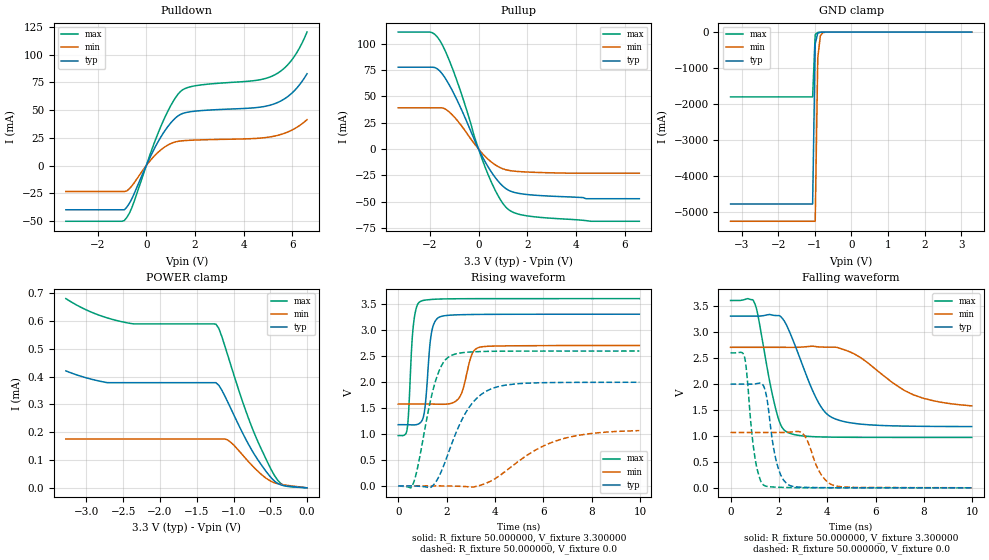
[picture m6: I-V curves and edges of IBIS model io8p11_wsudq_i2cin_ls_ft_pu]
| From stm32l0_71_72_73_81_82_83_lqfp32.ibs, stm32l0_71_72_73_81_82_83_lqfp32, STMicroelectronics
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|   Model io8p11_wsudq_i2cin_ls_ft_pu
[Model]  io8p11_wsudq_i2cin_ls_ft_pu
Model_type I/O
Polarity   Non-Inverting
Enable   Active-Low
Vinl =   0.990000V
Vinh =   2.310000V
Vmeas =  1.650000V
Cref =   50.000000pF
Rref =   100.000000M
Vref =   0.0V
C_comp   3.020400pF   2.988300pF   3.054500pF
[Temperature Range]   25.000000   0.125000k   -40.000000
[Pullup Reference]   3.300000V   2.700000V   3.600000V
[Pulldown Reference]   0.0V   0.0V   0.0V
[POWER Clamp Reference]   3.300000V   2.700000V   3.600000V
[GND Clamp Reference]   0.0V   0.0V   0.0V
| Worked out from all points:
|   slope of the pulldown table from 0 to 0.495 V, typ, clamps not added: 22.6 ohm
|   slope of the pullup table from 0 to 0.495 V, typ, clamps not added: 23.9 ohm
|   GND clamp passes 1 mA (typ) near -0.64 V on its own axis
|   rising waveform, R_fixture 50.000000, V_fixture 3.300000: 20-80 % time 224ps typ, 370ps min, 185ps max; typ from 1.18 V to 3.3 V
|   rising waveform, R_fixture 50.000000, V_fixture 0.0: 20-80 % time 1.18ns typ, 2.2ns min, 709ps max; typ from 0.001 V to 1.99 V
|   falling waveform, R_fixture 50.000000, V_fixture 3.300000: 20-80 % time 1.13ns typ, 2.04ns min, 653ps max; typ from 3.3 V to 1.18 V
|   falling waveform, R_fixture 50.000000, V_fixture 0.0: 20-80 % time 415ps typ, 586ps min, 336ps max; typ from 1.99 V to 0.001 V
[Pulldown]
|Voltage   I(typ)   I(min)   I(max)
-3.3V     -39.83mA   -23.37mA   -50.2mA
-900mV    -39.83mA   -23.37mA   -49.52mA
-600mV    -30.28mA   -18.59mA   -38.45mA
100mV     4.867mA    2.821mA    6.48mA
600mV     25.85mA    14.17mA    35.39mA
1V        38.33mA    19.81mA    53.88mA
1.4V      46.1mA     22.18mA    66.72mA
2V        49.07mA    23.02mA    71.93mA
4.4V      52.05mA    24.38mA    76.53mA
5.2V      55.25mA    26.31mA    81.02mA
6V        65.78mA    32.24mA    95.96mA
6.6V      82.83mA    41.41mA    120.4mA
[Pullup]
|Voltage   I(typ)   I(min)   I(max)
-3.3V     77.64mA    39.15mA    111mA
-2V       77.64mA    39.15mA    111mA
-1.6V     74.25mA    39.15mA    103.3mA
-1.3V     64.67mA    37mA       89.48mA
-900mV    47.24mA    27.86mA    65.53mA
-200mV    10.44mA    5.971mA    13.84mA
300mV     -13.29mA   -7.65mA    -18.99mA
800mV     -30.32mA   -16.54mA   -44.19mA
1.2V      -38.62mA   -20mA      -56.79mA
1.6V      -41.75mA   -21.17mA   -61.39mA
2.5V      -43.99mA   -22.16mA   -64.64mA
6.6V      -47mA      -22.8mA    -68.4mA
[GND_clamp]
|Voltage   I(typ)   I(min)   I(max)
-3.3V     -4.766A    -5.244A    -1.797A
-1.06V    -4.766A    -5.244A    -1.797A
-990mV    -326.6mA   -5.244A    -67.9mA
-920mV    -28.92mA   -722.1mA   -10.96mA
-850mV    -6.612mA   -104.2mA   -6.532mA
-780mV    -3.464mA   -17.27mA   -4.209mA
-500mV    -57.88uA   -167.8uA   -34.02uA
3.28V     0A         0A         0A
[POWER_clamp]
|Voltage   I(typ)   I(min)   I(max)
-3.28V    420.5uA    175.8uA    680.6uA
-2.72V    378.4uA    175.8uA    611.4uA
-2.4V     378.3uA    175.8uA    591.2uA
-1.24V    378.3uA    175.8uA    588.9uA
-1.2V     368.9uA    175.8uA    573.6uA
-1.08V    309.6uA    172.2uA    478.3uA
-920mV    220.5uA    131.5uA    344.5uA
-760mV    139.7uA    83.77uA    224.7uA
-480mV    33.95uA    22.2uA     61.82uA
-400mV    15.86uA    14.74uA    27.74uA
-320mV    8.147uA    10.83uA    9.34uA
0V        0A         0A         0A
[Ramp]
| variable   typ   min   max
dV/dt_r  1.19396/1.18030n   0.61121/2.08464n   1.55517/0.70833n
dV/dt_f  1.27116/1.13021n   0.59088/1.81656n   1.57796/0.65123n
R_load = 50.000000
[Rising Waveform]
R_fixture= 50.000000
V_fixture= 3.300000
V_fixture_min= 2.700000
V_fixture_max= 3.600000
|time   V(typ)   V(min)   V(max)
0s        1.178V     1.575V     968.8mV
360.4ps   1.177V     1.575V     1.068V
620.6ps   1.174V     1.575V     3.06V
920.9ps   1.218V     1.575V     3.547V
1.101ns   1.486V     1.575V     3.57V
1.381ns   2.958V     1.574V     3.584V
1.702ns   3.245V     1.571V     3.591V
2.503ns   3.289V     1.684V     3.597V
3.363ns   3.296V     2.665V     3.599V
9.97ns    3.3V       2.7V       3.6V
[Rising Waveform]
R_fixture= 50.000000
V_fixture= 0.0
V_fixture_min= 0.0
V_fixture_max= 0.0
|time   V(typ)   V(min)   V(max)
0s        1.058mV    1.825mV    441uV
620.6ps   350.3uV    1.809mV    45.69mV
800.8ps   -3.399mV   1.818mV    353.3mV
1.502ns   43.96mV    1.995mV    1.951V
1.802ns   303mV      1.642mV    2.322V
2.142ns   722mV      -583.6uV   2.495V
2.983ns   1.544V     -19.39mV   2.574V
3.924ns   1.88V      119mV      2.588V
6.486ns   1.988V     860.5mV    2.592V
9.97ns    1.993V     1.064V     2.593V
[Falling Waveform]
R_fixture= 50.000000
V_fixture= 3.300000
V_fixture_min= 2.700000
V_fixture_max= 3.600000
|time   V(typ)   V(min)   V(max)
0s        3.3V       2.7V       3.6V
981ps     3.3V       2.7V       3.563V
1.862ns   3.311V     2.7V       1.527V
2.082ns   3.287V     2.7V       1.203V
2.322ns   3.119V     2.7V       1.075V
3.504ns   1.758V     2.716V     981.9mV
4.204ns   1.35V      2.702V     974.3mV
5.145ns   1.238V     2.566V     970.8mV
7.568ns   1.184V     1.785V     969mV
9.97ns    1.178V     1.575V     968.8mV
[Falling Waveform]
R_fixture= 50.000000
V_fixture= 0.0
V_fixture_min= 0.0
V_fixture_max= 0.0
|time   V(typ)   V(min)   V(max)
0s        1.993V     1.064V     2.593V
580.6ps   1.992V     1.064V     2.51V
1.001ns   1.996V     1.064V     603.1mV
1.381ns   1.94V      1.064V     48.35mV
1.922ns   458.9mV    1.064V     12.59mV
2.462ns   43.19mV    1.071V     5.273mV
3.043ns   9.976mV    1.014V     2.655mV
3.664ns   5.028mV    317.7mV    1.736mV
4.304ns   3.307mV    40.36mV    1.233mV
9.97ns    1.058mV    1.825mV    441uV
